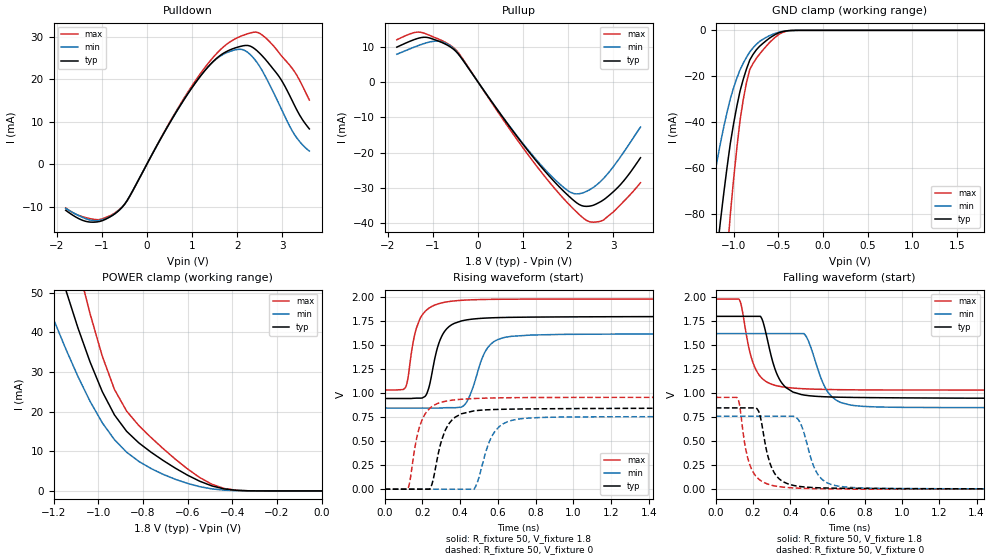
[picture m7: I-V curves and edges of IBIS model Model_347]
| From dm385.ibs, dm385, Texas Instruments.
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| Model based on original model for BCSHTLTCSCDDVPBFZ_SSDHV
|   Sub model SR00_7MA_PADP_10PER_1P8
[model]   Model_347
|[Description]  [1.8V-3-STATE-NOTERM-FASTEST:7MA, IND, 10%]
|   Fastest slew rate (SR[1:0] = "00"), 1.14 * RExt = 0.875 * Iout
|   (I[2:0] = "010"), 7mA nominal with Rext = 50R,ODT off (ODT[1:0]
|   = "00") CMOS mode,Industrial temperature range (-40C to 125C,
|   25C nominal),10% power supply tolerance
|[Input Load]   NOTERM
|[Output Drive] FASTEST:7MA
|Voltage   1.8V
|Mode   3-STATE
Model_type   3-state
Polarity   Non-Inverting
Enable   Active-Low
Cref =  15pF
Rref =  100.0000M
Vref =  0V
Vmeas =  0.9
C_comp   1.851324p   1.663768p   1.973575p
[Temperature Range]   25   125   -40
[Voltage Range]   1.8   1.62   1.98
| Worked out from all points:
|   slope of the pulldown table from 0 to 0.27 V, typ, clamps not added: 51.1 ohm
|   slope of the pullup table from 0 to 0.27 V, typ, clamps not added: 54.4 ohm
|   GND clamp passes 1 mA (typ) near -0.49 V on its own axis
|   POWER clamp passes 1 mA (typ) near -0.47 V on its own axis
|   rising waveform, R_fixture 50, V_fixture 1.8: 20-80 % time 70.8ps typ, 85.7ps min, 63ps max; typ from 0.944 V to 1.8 V
|   rising waveform, R_fixture 50, V_fixture 0: 20-80 % time 73.9ps typ, 81.5ps min, 67.1ps max; typ from 0 V to 0.842 V
|   falling waveform, R_fixture 50, V_fixture 1.8: 20-80 % time 81.8ps typ, 92.8ps min, 73.2ps max; typ from 1.8 V to 0.946 V
|   falling waveform, R_fixture 50, V_fixture 0: 20-80 % time 66.4ps typ, 77.9ps min, 61.1ps max; typ from 0.846 V to 0.004 V
[POWER_clamp]
-1.8V     194.9mA    137.1mA    262.8mA
-1.236V   68.49mA    48.51mA    92.67mA
-1.145V   50.76mA    35.86mA    69.65mA
-1.127V   47.56mA    33.54mA    65.34mA
-1.055V   35.4mA     24.69mA    48.69mA
-981.8mV  25.06mA    17.2mA     34.01mA
-927.3mV  19.17mA    12.93mA    25.61mA
-872.7mV  15.03mA    9.767mA    20.12mA
-818.2mV  12.12mA    7.45mA     16.5mA
-654.5mV  5.738mA    2.93mA     8.003mA
-436.4mV  508.2uA    199.4uA    613uA
0V        2.273nA    15.95nA    16.67nA
[Pulldown]
-1.8V     -10.87mA   -10.42mA   -10.31mA
-1.145V   -13.64mA   -13.33mA   -13.03mA
-545.5mV  -10.12mA   -10.08mA   -10.04mA
545.5mV   10.39mA    10.38mA    10.59mA
1.091V    19.34mA    19.35mA    19.85mA
1.527V    24.71mA    24.62mA    25.8mA
1.964V    27.34mA    26.87mA    29.49mA
2.291V    27.74mA    25.74mA    30.83mA
2.618V    24.71mA    20.75mA    29.8mA
2.945V    20.32mA    13.73mA    25.93mA
3.218V    14.95mA    7.852mA    22.54mA
3.6V      8.27mA     3.068mA    15.06mA
[Pullup]
-1.8V     9.872mA    7.849mA    11.96mA
-1.309V   12.43mA    10.38mA    14.13mA
-927.3mV  11.82mA    11.58mA    12.42mA
-600mV    9.811mA    10.09mA    10.26mA
-381.8mV  7.028mA    7.03mA     7.372mA
1.2V      -20.91mA   -20.59mA   -22.11mA
1.745V    -28.92mA   -28.09mA   -30.81mA
2.127V    -33.58mA   -31.56mA   -36.06mA
2.455V    -35.14mA   -30.6mA    -39.44mA
2.727V    -33.77mA   -27.97mA   -39.32mA
3.164V    -28.92mA   -21.05mA   -34.62mA
3.6V      -21.41mA   -12.75mA   -28.48mA
[GND_clamp]
-1.8V     -346.1mA   -209.3mA   -568.3mA
-1.327V   -149.7mA   -89.03mA   -250.9mA
-1.291V   -135.6mA   -80.47mA   -227.5mA
-1.145V   -82.35mA   -48.67mA   -137.7mA
-1.073V   -59.44mA   -35.55mA   -97.96mA
-1.036V   -49.1mA    -29.72mA   -79.9mA
-927.3mV  -26.31mA   -17.11mA   -38.99mA
-854.5mV  -16.67mA   -11.64mA   -22.56mA
-818.2mV  -12.86mA   -9.351mA   -16.98mA
-672.7mV  -5.705mA   -3.913mA   -8.624mA
-381.8mV  -120.4uA   -129uA     -167.4uA
1.8V      2.273nA    454nA      6.646nA
[Ramp]
dV/dt_f 0.52134932/82.708176p 0.47544485/94.59343p  0.57395421/73.31721p
dV/dt_r  0.5138886/74.772403p 0.46511205/82.582845p 0.57849377/67.072951p
R_load = 50
[Rising Waveform]
R_fixture = 50
V_fixture = 1.8
V_fixture_min = 1.62
V_fixture_max = 1.98
0s        944.4mV    844.3mV    1.033V
110.5ps   944.4mV    844.3mV    1.058V
165ps     947.8mV    844.3mV    1.655V
214.1ps   965.9mV    844.3mV    1.851V
295.1ps   1.56V      845.1mV    1.936V
340.3ps   1.692V     849.1mV    1.954V
421.8ps   1.758V     874.2mV    1.969V
533.5ps   1.782V     1.435V     1.976V
624.4ps   1.788V     1.575V     1.978V
1.787ns   1.798V     1.616V     1.98V
[Rising Waveform]
R_fixture = 50
V_fixture = 0
V_fixture_min = 0
V_fixture_max = 0
0s        0V         0V         0V
121.7ps   0V         0V         0V
182.2ps   0V         0V         629.6mV
239.8ps   0V         0V         842.9mV
301.7ps   507.3mV    0V         906.1mV
356.4ps   719.3mV    0V         926.7mV
473.8ps   815.7mV    0V         944.1mV
570.8ps   828.9mV    559.8mV    949.7mV
673.4ps   833.7mV    716.3mV    952.8mV
1.839ns   842.5mV    755mV      955.9mV
[Falling Waveform]
R_fixture = 50
V_fixture = 1.8
V_fixture_min = 1.62
V_fixture_max = 1.98
0s        1.799V     1.62V      1.979V
128.5ps   1.799V     1.62V      1.967V
187.7ps   1.799V     1.62V      1.393V
240.3ps   1.799V     1.62V      1.171V
315.6ps   1.264V     1.62V      1.083V
376.3ps   1.058V     1.62V      1.06V
474.5ps   979.7mV    1.62V      1.045V
587.2ps   961.8mV    1.058V     1.038V
676.2ps   957mV      898.8mV    1.035V
1.787ns   946mV      849mV      1.032V
[Falling Waveform]
R_fixture = 50
V_fixture = 0
V_fixture_min = 0
V_fixture_max = 0
0s        846.1mV    759.8mV    955.4mV
118.7ps   846.1mV    759.8mV    942mV
170.3ps   846.1mV    759.8mV    335.1mV
221.3ps   838.1mV    759.8mV    122.5mV
297.3ps   237.6mV    759.8mV    42.31mV
341.3ps   105.6mV    759.8mV    25.87mV
442.5ps   30.49mV    725.8mV    10.61mV
535.1ps   15.73mV    198mV      5.658mV
627.6ps   10.77mV    44.22mV    3.277mV
1.839ns   3.836mV    3.923mV    0V
